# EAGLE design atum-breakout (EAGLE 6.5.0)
AUTHOR: Brad Campbell; REV: A; TITLE: Atum Breakout
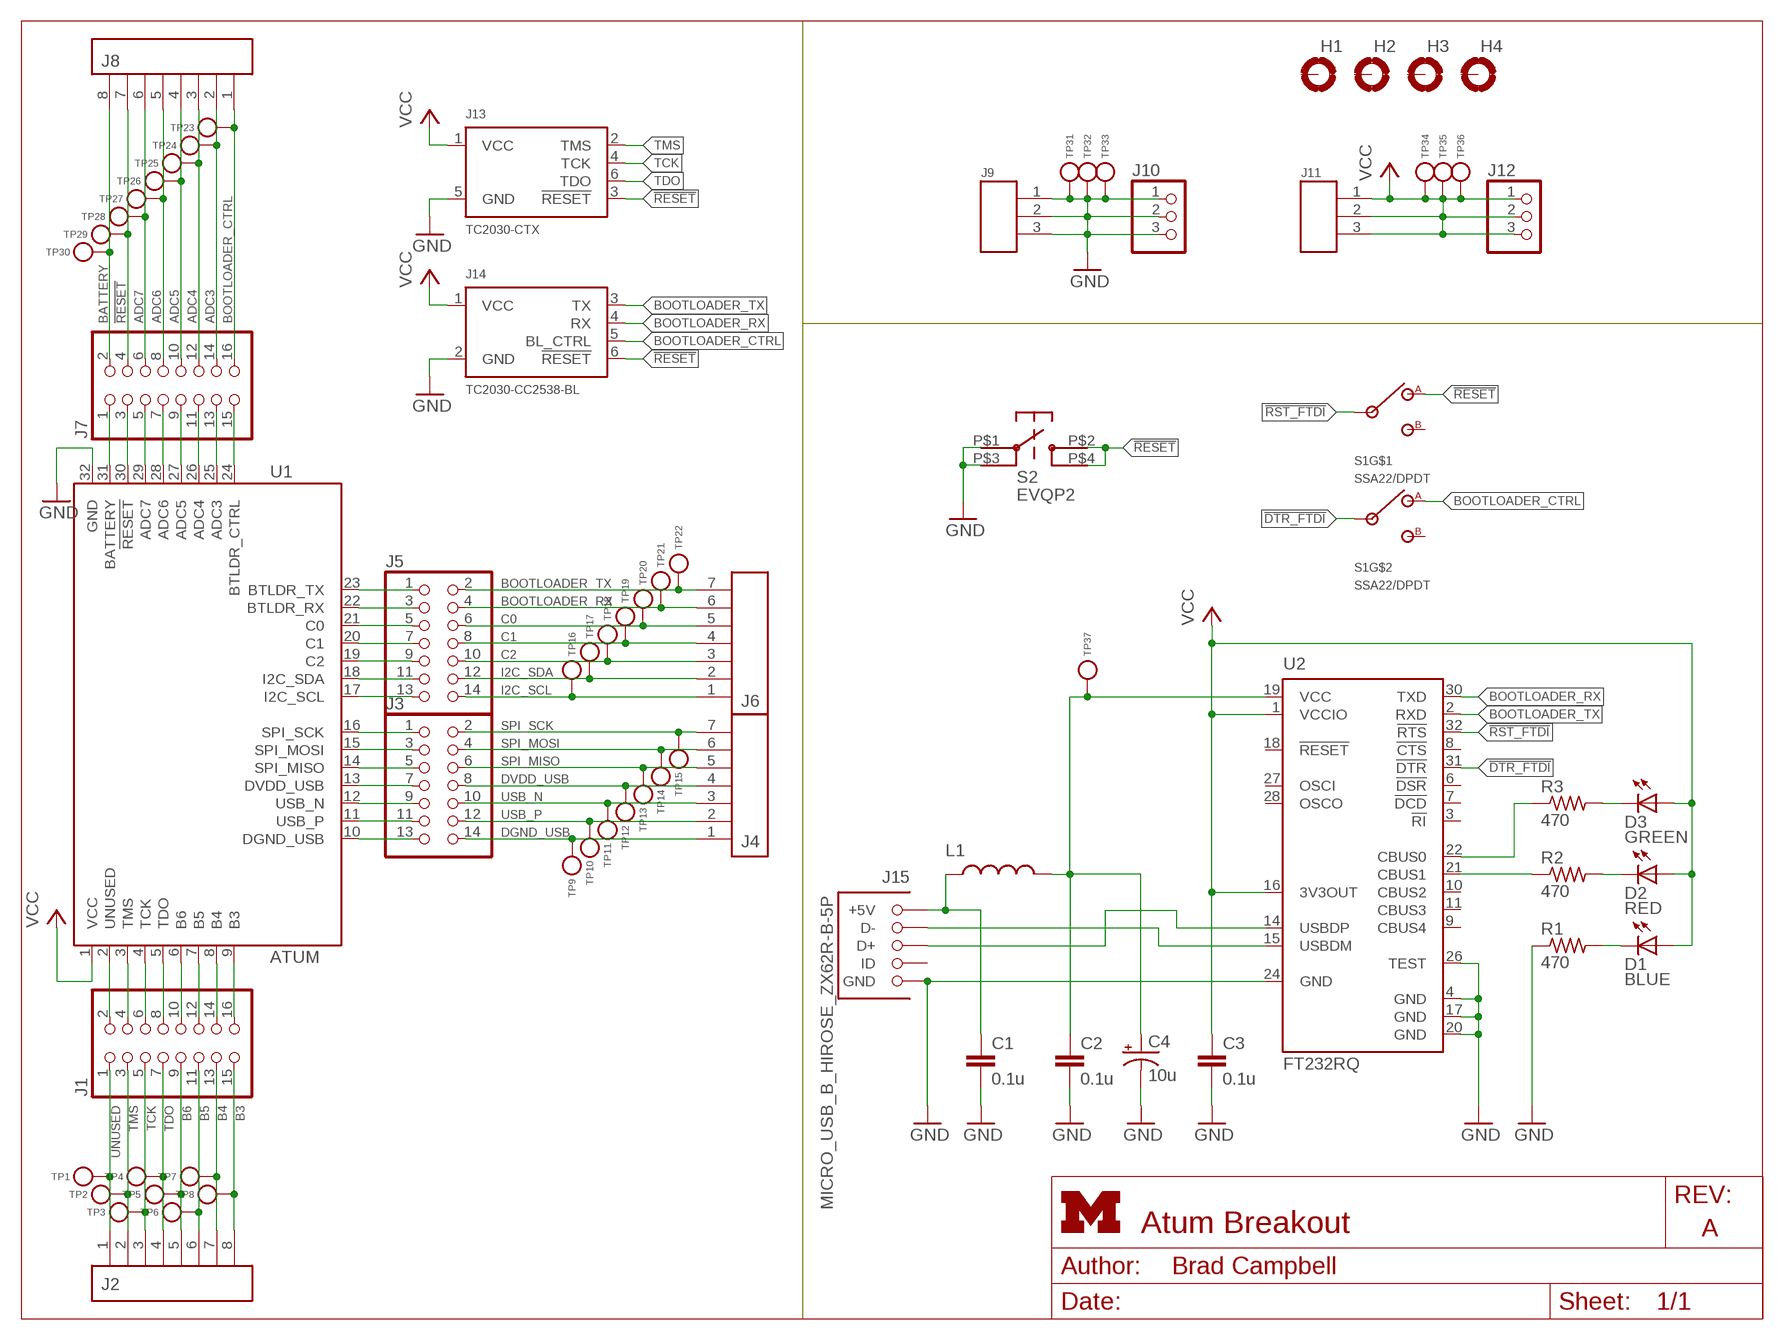
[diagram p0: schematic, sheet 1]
FRAME1 (LETTER_L): HEIGHT: 8.5in; WIDTH: 11in

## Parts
C1  0.1u  C-EUC0603  [C0603]
C2  0.1u  C-EUC0603  [C0603]
C3  0.1u  C-EUC0603  [C0603]
C4  10u  CAP_POL1206  [EIA3216]
D1  BLUE  LED0603  [LED-0603]
D2  RED  LED0603  [LED-0603]
D3  GREEN  LED0603  [LED-0603]
H1  MOUNT-PAD-ROUND3.2  [3,2-PAD]
H2  MOUNT-PAD-ROUND3.2  [3,2-PAD]
H3  MOUNT-PAD-ROUND3.2  [3,2-PAD]
H4  MOUNT-PAD-ROUND3.2  [3,2-PAD]
J1  PINHD-2X8  [2X08]
J2  SCREW-TERMINAL_8_0.100  [CONN_BLOCK_8]
J3  PINHD-2X7  [2X07]
J4  SCREW-TERMINAL_7_0.100  [CONN_BLOCK_7]
J5  PINHD-2X7  [2X07]
J6  SCREW-TERMINAL_7_0.100  [CONN_BLOCK_7]
J7  PINHD-2X8  [2X08]
J8  SCREW-TERMINAL_8_0.100  [CONN_BLOCK_8]
J9  SCREW-TERMINAL_3_0.100  [CONN_BLOCK_3]
J10  PINHD-1X3  [1X03]
J11  SCREW-TERMINAL_3_0.100  [CONN_BLOCK_3]
J12  PINHD-1X3  [1X03]
J13  TC2030-CTX  [TC2030-IDC]
J14  TC2030-CC2538-BL  [TC2030-IDC]
J15  MICRO_USB_B_HIROSE_ZX62R-B-5P  [USB_MICRO_B-HIROSE-ZX62R-B-5P]
L1  INDUCTOR0603  [0603]
R1  470  R-US_R0603  [R0603]
R2  470  R-US_R0603  [R0603]
R3  470  R-US_R0603  [R0603]
S1  SSA22/DPDT  [SSA22/DPDT]
S2  EVQP2  [EVQP2]
TP1  TEST_POINT_0.040IN  [TESTPOINT_0.040IN]
TP2  TEST_POINT_0.040IN  [TESTPOINT_0.040IN]
TP3  TEST_POINT_0.040IN  [TESTPOINT_0.040IN]
TP4  TEST_POINT_0.040IN  [TESTPOINT_0.040IN]
TP5  TEST_POINT_0.040IN  [TESTPOINT_0.040IN]
TP6  TEST_POINT_0.040IN  [TESTPOINT_0.040IN]
TP7  TEST_POINT_0.040IN  [TESTPOINT_0.040IN]
TP8  TEST_POINT_0.040IN  [TESTPOINT_0.040IN]
TP9  TEST_POINT_0.040IN  [TESTPOINT_0.040IN]
TP10  TEST_POINT_0.040IN  [TESTPOINT_0.040IN]
TP11  TEST_POINT_0.040IN  [TESTPOINT_0.040IN]
TP12  TEST_POINT_0.040IN  [TESTPOINT_0.040IN]
TP13  TEST_POINT_0.040IN  [TESTPOINT_0.040IN]
TP14  TEST_POINT_0.040IN  [TESTPOINT_0.040IN]
TP15  TEST_POINT_0.040IN  [TESTPOINT_0.040IN]
TP16  TEST_POINT_0.040IN  [TESTPOINT_0.040IN]
TP17  TEST_POINT_0.040IN  [TESTPOINT_0.040IN]
TP18  TEST_POINT_0.040IN  [TESTPOINT_0.040IN]
TP19  TEST_POINT_0.040IN  [TESTPOINT_0.040IN]
TP20  TEST_POINT_0.040IN  [TESTPOINT_0.040IN]
TP21  TEST_POINT_0.040IN  [TESTPOINT_0.040IN]
TP22  TEST_POINT_0.040IN  [TESTPOINT_0.040IN]
TP23  TEST_POINT_0.040IN  [TESTPOINT_0.040IN]
TP24  TEST_POINT_0.040IN  [TESTPOINT_0.040IN]
TP25  TEST_POINT_0.040IN  [TESTPOINT_0.040IN]
TP26  TEST_POINT_0.040IN  [TESTPOINT_0.040IN]
TP27  TEST_POINT_0.040IN  [TESTPOINT_0.040IN]
TP28  TEST_POINT_0.040IN  [TESTPOINT_0.040IN]
TP29  TEST_POINT_0.040IN  [TESTPOINT_0.040IN]
TP30  TEST_POINT_0.040IN  [TESTPOINT_0.040IN]
TP31  TEST_POINT_0.040IN  [TESTPOINT_0.040IN]
TP32  TEST_POINT_0.040IN  [TESTPOINT_0.040IN]
TP33  TEST_POINT_0.040IN  [TESTPOINT_0.040IN]
TP34  TEST_POINT_0.040IN  [TESTPOINT_0.040IN]
TP35  TEST_POINT_0.040IN  [TESTPOINT_0.040IN]
TP36  TEST_POINT_0.040IN  [TESTPOINT_0.040IN]
TP37  TEST_POINT_0.040IN  [TESTPOINT_0.040IN]
U1  ATUM  [ATUM]
U2  FT232RQ  [QFN32]

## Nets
!DTR_FTDI: S1.COM2 U2.31(!DTR)
!RESET: J7.3 J7.4 J8.7 J13.3(!RESET) J14.6(!RESET) S1.A1 S2.P$2 S2.P$4 TP29.TESTPOINT U1.30(!RESET)
!RST_FTDI: S1.COM1 U2.32(!RTS)
ADC3: J7.13 J7.14 J8.2 TP24.TESTPOINT U1.25(ADC3)
ADC4: J7.11 J7.12 J8.3 TP25.TESTPOINT U1.26(ADC4)
ADC5: J7.9 J7.10 J8.4 TP26.TESTPOINT U1.27(ADC5)
ADC6: J7.7 J7.8 J8.5 TP27.TESTPOINT U1.28(ADC6)
ADC7: J7.5 J7.6 J8.6 TP28.TESTPOINT U1.29(ADC7)
B3: J1.15 J1.16 J2.8 TP8.TESTPOINT U1.9(B3)
B4: J1.13 J1.14 J2.7 TP7.TESTPOINT U1.8(B4)
B5: J1.11 J1.12 J2.6 TP6.TESTPOINT U1.7(B5)
B6: J1.9 J1.10 J2.5 TP5.TESTPOINT U1.6(B6)
BATTERY: J7.1 J7.2 J8.8 TP30.TESTPOINT U1.31(BATTERY)
BOOTLOADER_CTRL: J7.15 J7.16 J8.1 J14.5(BL_CTRL) S1.A2 TP23.TESTPOINT U1.24(BTLDR_CTRL)
BOOTLOADER_RX: J5.3 J5.4 J6.6 J14.4(RX) TP21.TESTPOINT U1.22(BTLDR_RX) U2.30(TXD)
BOOTLOADER_TX: J5.1 J5.2 J6.7 J14.3(TX) TP22.TESTPOINT U1.23(BTLDR_TX) U2.2(RXD)
C0: J5.5 J5.6 J6.5 TP20.TESTPOINT U1.21(C0)
C1: J5.7 J5.8 J6.4 TP19.TESTPOINT U1.20(C1)
C2: J5.9 J5.10 J6.3 TP18.TESTPOINT U1.19(C2)
DGND_USB: J3.13 J3.14 J4.1 TP9.TESTPOINT U1.10(DGND_USB)
DVDD_USB: J3.7 J3.8 J4.4 TP12.TESTPOINT U1.13(DVDD_USB)
GND: C1.2 C2.2 C3.2 C4.C(-) J9.1 J9.2 J9.3 J10.1 J10.2 J10.3 J13.5(GND) J14.2(GND) J15.5(GND) R1.1 S2.P$1 S2.P$3 TP31.TESTPOINT TP32.TESTPOINT TP33.TESTPOINT U1.32(GND) U2.4(GND) U2.17(GND) U2.20(GND) U2.24(GND) U2.26(TEST)
I2C_SCL: J5.13 J5.14 J6.1 TP16.TESTPOINT U1.17(I2C_SCL)
I2C_SDA: J5.11 J5.12 J6.2 TP17.TESTPOINT U1.18(I2C_SDA)
N$1: R3.1 U2.22(CBUS0)
N$2: D2.C R2.2
N$3: J15.2(D-) U2.15(USBDM)
N$4: J15.3(D+) U2.14(USBDP)
N$5: R2.1 U2.21(CBUS1)
N$6: C2.1 C4.A(+) L1.2 TP37.TESTPOINT U2.19(VCC)
N$7: D3.C R3.2
N$8: D1.C R1.2
SPI_MISO: J3.5 J3.6 J4.5 TP13.TESTPOINT U1.14(SPI_MISO)
SPI_MOSI: J3.3 J3.4 J4.6 TP14.TESTPOINT U1.15(SPI_MOSI)
SPI_SCK: J3.1 J3.2 J4.7 TP15.TESTPOINT U1.16(SPI_SCK)
TCK: J1.5 J1.6 J2.3 J13.4(TCK) TP3.TESTPOINT U1.4(TCK)
TDO: J1.7 J1.8 J2.4 J13.6(TDO) TP4.TESTPOINT U1.5(TDO)
TMS: J1.3 J1.4 J2.2 J13.2(TMS) TP2.TESTPOINT U1.3(TMS)
UNUSED: J1.1 J1.2 J2.1 TP1.TESTPOINT U1.2(UNUSED)
USB5V: C1.1 J15.1(+5V) L1.1
USB_N: J3.9 J3.10 J4.3 TP11.TESTPOINT U1.12(USB_N)
USB_P: J3.11 J3.12 J4.2 TP10.TESTPOINT U1.11(USB_P)
VCC: C3.1 D1.A D2.A D3.A J11.1 J11.2 J11.3 J12.1 J12.2 J12.3 J13.1(VCC) J14.1(VCC) TP34.TESTPOINT TP35.TESTPOINT TP36.TESTPOINT U1.1(VCC) U2.1(VCCIO) U2.16(3V3OUT)
Unconnected: H1.B3,2(MOUNT) H2.B3,2(MOUNT) H3.B3,2(MOUNT) H4.B3,2(MOUNT) J15.4(ID) S1.B1 S1.B2 U2.3(!RI) U2.6(!DSR) U2.7(!DCD) U2.8(!CTS) U2.9(CBUS4) U2.10(CBUS2) U2.11(CBUS3) U2.18(!RESET) U2.27(OSCI) U2.28(OSCO)

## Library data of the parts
C1-C3 = rcl:C-EU: CAPACITOR, European symbol; DIGIKEY: 445-1316-1-ND
C4 = SparkFun:CAP_POL: Capacitor Polarized; DIGIKEY: 478-1655-1-ND
D1-D3 = SparkFun:LED: LEDs
H1-H4 = holes:MOUNT-PAD-ROUND: MOUNTING PAD, round
J1 J7 = pinhead:PINHD-2X8: PIN HEADER; DIGIKEY: 609-3364-ND; MOUSER: 649-68602-116HLF; NEWARK: 20M2833
J2 J8 = headers:SCREW-TERMINAL_8_0.100: 8x 0.100 in screw terminal block; DIGIKEY: 277-1279-ND
J3 J5 = pinhead:PINHD-2X7: PIN HEADER; DIGIKEY: 609-3491-ND; MOUSER: 649-67996-114HLF; NEWARK: 30M1973
J4 J6 = headers:SCREW-TERMINAL_7_0.100: 7x 0.100 in screw terminal block; DIGIKEY: 277-1278-ND
J9 J11 = headers:SCREW-TERMINAL_3_0.100: 3x 0.100 in screw terminal block; DIGIKEY: 277-1274-ND
J10 J12 = pinhead:PINHD-1X3: PIN HEADER
J13 = connector:TC2030-CTX: Tag Connect footprint for ARM JTAG. 10 pin ARM Cortex Debug Connector.
J14 = connector:TC2030-CC2538-BL: Tag connect programmer for the CC2538 bootloader. The RX/TX switch happens on the programmer board, so when using this connect the TX pin to the TX pin on the CC2538 and same for the RX.
J15 = connector:MICRO_USB_B_HIROSE_ZX62R-B-5P: USB Micro B Connector Rounded side is up.; DIGIKEY: H11574CT-ND; MOUSER: 798-ZX62R-B-5P; NEWARK: 69W0714
L1 = SparkFun:INDUCTOR: Inductors; DIGIKEY: 240-2373-1-ND
R1-R3 = rcl:R-US_: RESISTOR, American symbol
S1 = switches:SSA22/DPDT: SW SLIDE DPDT 2POS SSA SER 30V; DIGIKEY: 450-1604-ND; MOUSER: 506-SSA22; NEWARK: 50F5561
S2 = berkeley-epic:EVQP2; DIGIKEY: P11084SCT-ND; MOUSER: 667-EVQ-P2K02Q
TP1-TP37 = headers:TEST_POINT_0.040IN: 0.040in Test Point; DIGIKEY: 5001K-ND
U1 = atum:ATUM: Atum sensorboard prototyping module.
U2 = ftdichip:FT232R: Source: http://www.ftdichip.com/Documents/DataSheets/DS_FT232R_v104.pdf; DIGIKEY: 768-1008-1-ND; MPN: FT232RQ; OC_FARNELL: 1146033; OC_NEWARK: 91K9919

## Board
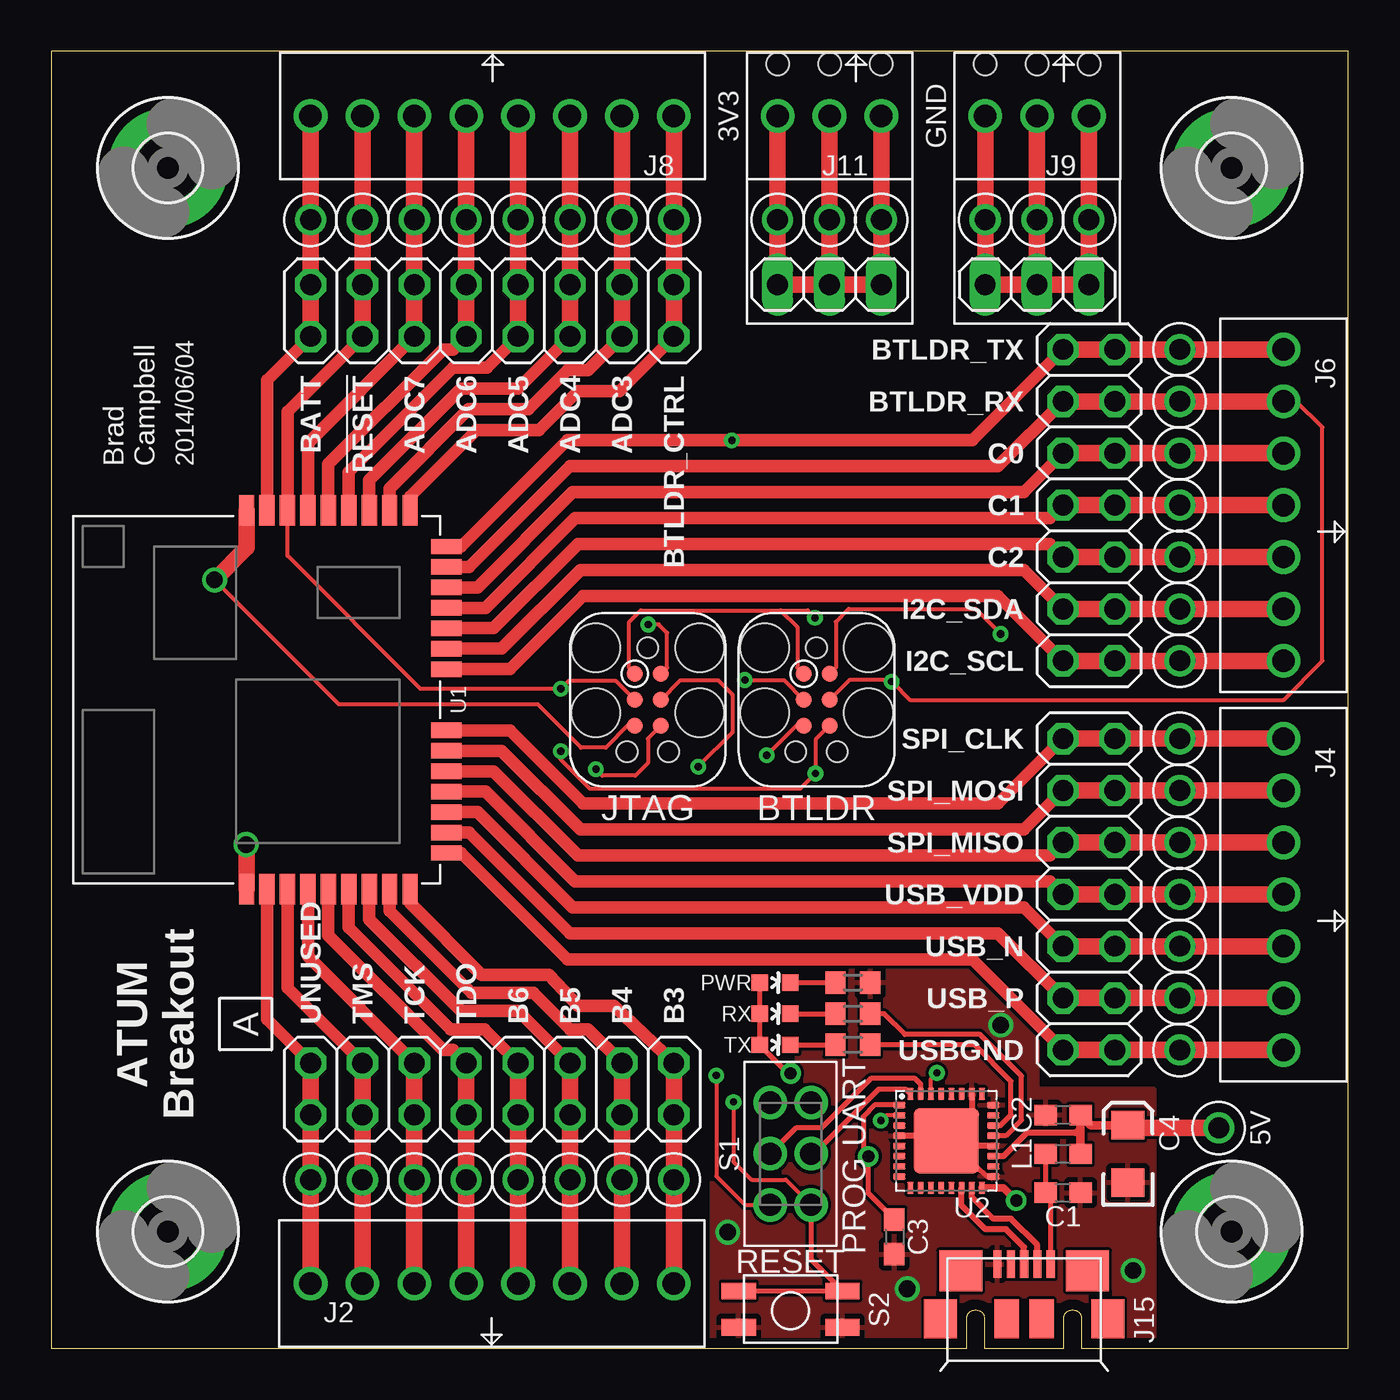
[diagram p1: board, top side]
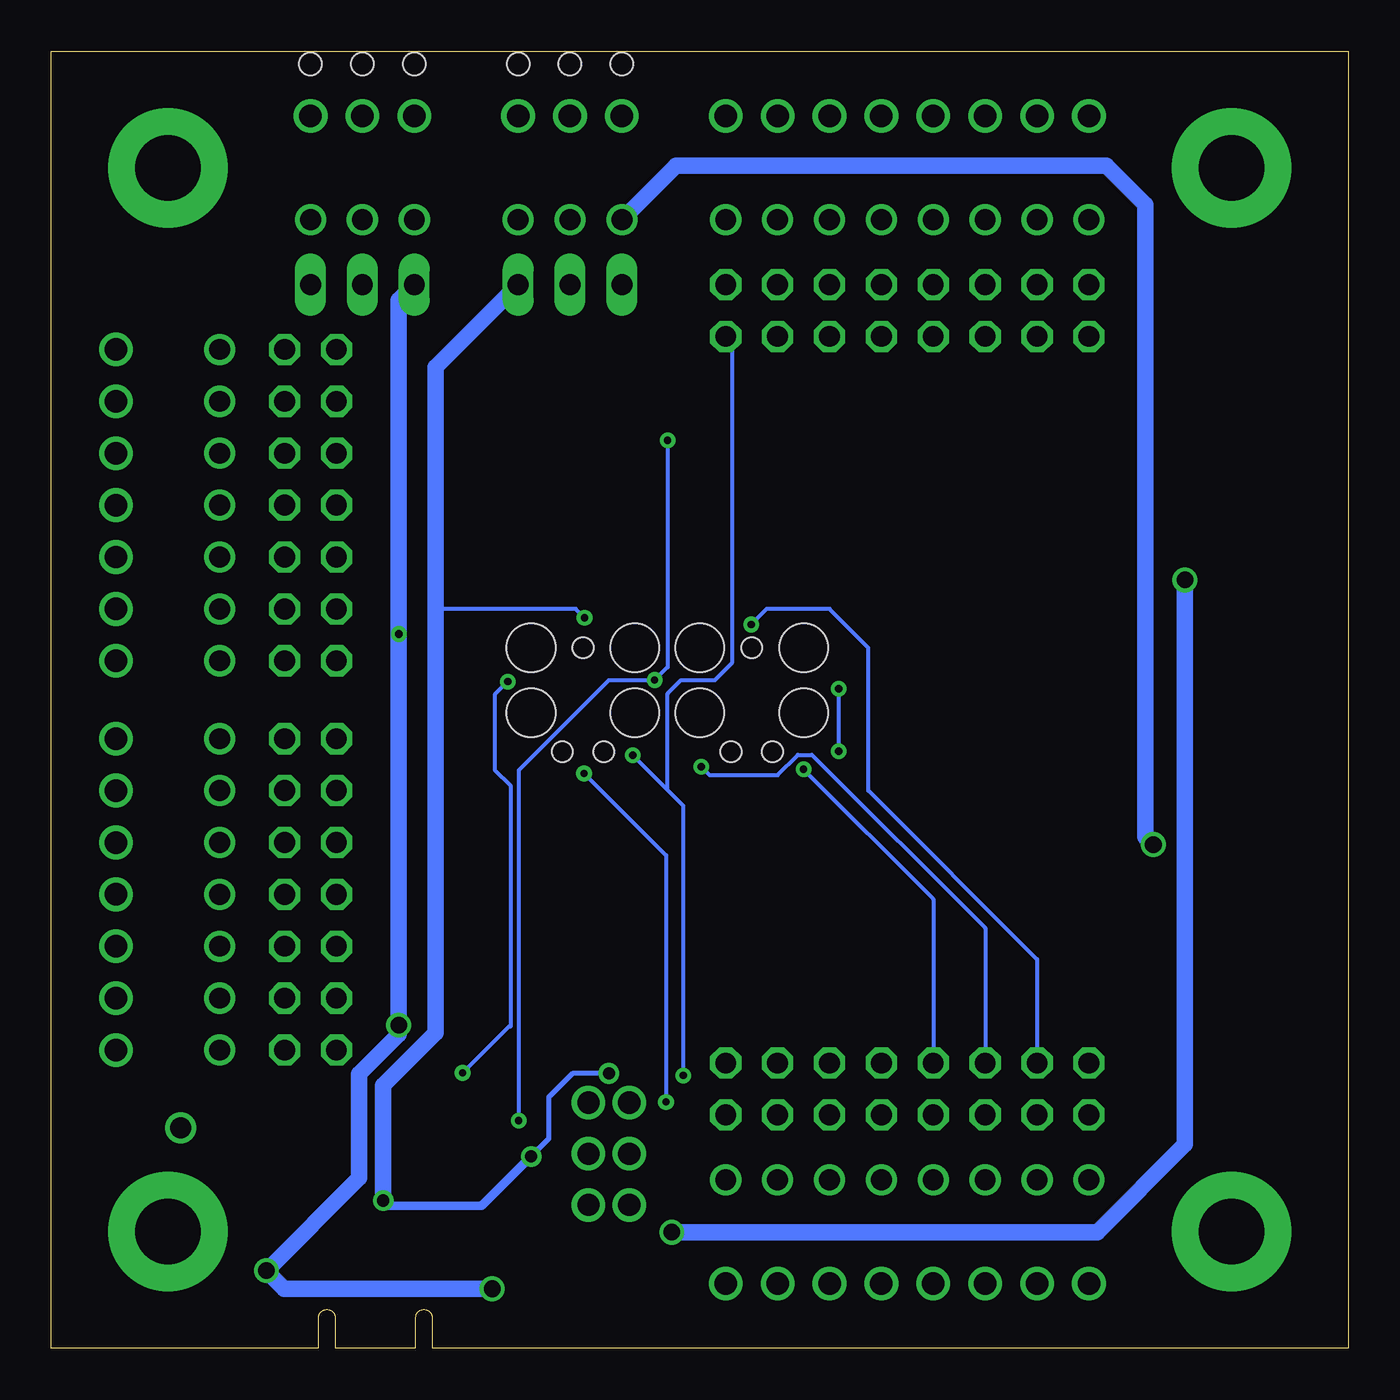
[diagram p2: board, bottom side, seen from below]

Size 63.5 x 63.5 mm. Coordinates in mm from the lower left corner, seen from the top.
Outline: 52.7,0 63.5,0 63.5,63.5 0,63.5 0,0 42.55,0
Copper layers (1*16): Top 0.0178mm / dielectric 59mil / Bottom 0.0178mm
Design rules "sunstone-2lyr_v1.0.0.3 *": minimum track width 6mil, minimum drill 14mil, track to track 6mil, track to pad 6mil, pad to pad 6mil, via to via 6mil, smd to smd 6mil, copper to edge 20mil, drill to drill 16mil, minimum pad ring 8mil, minimum via ring 8mil, stop-mask expansion 3mil, vias tented up to drill 40mil, thermal gap 10mil

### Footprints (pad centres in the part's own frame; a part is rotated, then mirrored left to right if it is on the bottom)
C0603 = smd 1.1 x 1: 1 -0.85,0; 2 0.85,0
EIA3216 = smd 1.4 x 1.6: A 1.4,0; C -1.4,0
LED-0603 = smd 0.8 x 0.8: A 0,-0.75; C 0,0.75
3,2-PAD = drill 3.2 pad 5.842: B3,2 0,0
2X08 = drill 1.016 octagon: 1 -8.89,-1.27; 2 -8.89,1.27; 3 -6.35,-1.27; 4 -6.35,1.27; 5 -3.81,-1.27; 6 -3.81,1.27; 7 -1.27,-1.27; 8 -1.27,1.27; 9 1.27,-1.27; 10 1.27,1.27; 11 3.81,-1.27; 12 3.81,1.27; 13 6.35,-1.27; 14 6.35,1.27; 15 8.89,-1.27; 16 8.89,1.27
CONN_BLOCK_8 = drill 1.1: 1 -8.89,0; 2 -6.35,0; 3 -3.81,0; 4 -1.27,0; 5 1.27,0; 6 3.81,0; 7 6.35,0; 8 8.89,0
2X07 = drill 1.016 octagon: 1 -7.62,-1.27; 2 -7.62,1.27; 3 -5.08,-1.27; 4 -5.08,1.27; 5 -2.54,-1.27; 6 -2.54,1.27; 7 0,-1.27; 8 0,1.27; 9 2.54,-1.27; 10 2.54,1.27; 11 5.08,-1.27; 12 5.08,1.27; 13 7.62,-1.27; 14 7.62,1.27
CONN_BLOCK_7 = drill 1.1: 1 -7.62,0; 2 -5.08,0; 3 -2.54,0; 4 0,0; 5 2.54,0; 6 5.08,0; 7 7.62,0
CONN_BLOCK_3 = drill 1.1: 1 -2.54,0; 2 0,0; 3 2.54,0 | hole 1.1: -2.54,-2.54; 0,-2.54; 2.54,-2.54
1X03 = drill 1.016 long: 1 -2.54,0; 2 0,0; 3 2.54,0
TC2030-IDC = smd 0.787 x 0.787: 1 -1.27,-0.635; 2 -1.27,0.635; 3 0,-0.635; 4 0,0.635; 5 1.27,-0.635; 6 1.27,0.635 | hole 2.375: -2.54,2.54; 0.635,2.54; 0.635,-2.54; -2.54,-2.54 | hole 1.016: -2.54,0; 2.54,1.016; 2.54,-1.016
USB_MICRO_B-HIROSE-ZX62R-B-5P = smd 0.4 x 1.35: 1 1.3,4.125; 2 0.65,4.125; 3 0,4.125; 4 -0.65,4.125; 5 -1.3,4.125 | smd 2.1 x 2: P$1 3.1,3.8; P$2 -3.1,3.8 | smd 1.6 x 1.9: P$3 -4.1,1.45; P$6 4.1,1.45 | smd 1.2 x 1.9: P$4 -0.85,1.45; P$5 0.85,1.45
0603 = smd 1.1 x 1: 1 -0.85,0; 2 0.85,0
R0603 = smd 1 x 1.1: 1 -0.85,0; 2 0.85,0
SSA22/DPDT = drill 1.092: A1 2.5,1; A2 2.5,-1; B1 -2.5,1; B2 -2.5,-1; COM1 0,1; COM2 0,-1
EVQP2 = smd 1.676 x 0.813: P$1 -2.54,-0.87; P$2 -2.54,0.908; P$3 2.54,-0.87; P$4 2.54,0.908
TESTPOINT_0.040IN = drill 1.016: TESTPOINT 0,0
ATUM = smd 0.754 x 1.5: 1 -9.479,-9.279; 2 -8.479,-9.279; 3 -7.479,-9.279; 4 -6.479,-9.279; 5 -5.479,-9.279; 6 -4.479,-9.279; 7 -3.479,-9.279; 8 -2.479,-9.279; 9 -1.479,-9.279; 24 -1.479,9.279; 25 -2.479,9.279; 26 -3.479,9.279; 27 -4.479,9.279; 28 -5.479,9.279; 29 -6.479,9.279; 30 -7.479,9.279; 31 -8.479,9.279; 32 -9.479,9.279 | smd 1.5 x 0.754: 10 0.3,-7.5; 11 0.3,-6.5; 12 0.3,-5.5; 13 0.3,-4.5; 14 0.3,-3.5; 15 0.3,-2.5; 16 0.3,-1.5; 17 0.3,1.5; 18 0.3,2.5; 19 0.3,3.5; 20 0.3,4.5; 21 0.3,5.5; 22 0.3,6.5; 23 0.3,7.5
QFN32 = smd 0.6 x 0.3: 1 -2.3,1.75; 2 -2.3,1.25; 3 -2.3,0.75; 4 -2.3,0.25; 5 -2.3,-0.25; 6 -2.3,-0.75; 7 -2.3,-1.25; 8 -2.3,-1.75; 17 2.3,-1.75; 18 2.3,-1.25; 19 2.3,-0.75; 20 2.3,-0.25; 21 2.3,0.25; 22 2.3,0.75; 23 2.3,1.25; 24 2.3,1.75 | smd 0.3 x 0.6: 9 -1.75,-2.3; 10 -1.25,-2.3; 11 -0.75,-2.3; 12 -0.25,-2.3; 13 0.25,-2.3; 14 0.75,-2.3; 15 1.25,-2.3; 16 1.75,-2.3; 25 1.75,2.3; 26 1.25,2.3; 27 0.75,2.3; 28 0.25,2.3; 29 -0.25,2.3; 30 -0.75,2.3; 31 -1.25,2.3; 32 -1.75,2.3 | smd 3.2 x 3.2: EXP 0,0

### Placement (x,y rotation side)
C1  49.53,7.62 0 top
C2  49.53,11.43 180 top
C3  41.27,5.46 270 top
C4  52.7,9.53 90 top
D1  35.43,17.91 270 top
D2  35.43,16.38 270 top
D3  35.43,14.86 270 top
H1  57.78,5.71 0 top
H2  5.71,5.71 0 top
H3  57.78,57.78 0 top
H4  5.71,57.78 0 top
J1  21.59,12.7 0 top
J2  21.59,3.17 0 top
J3  50.8,22.23 270 top
J4  60.33,22.23 90 top
J5  50.8,41.27 270 top
J6  60.33,41.27 90 top
J7  21.59,50.8 0 top
J8  21.59,60.33 180 top
J9  48.26,60.33 180 top
J10  48.26,52.07 0 top
J11  38.1,60.33 180 top
J12  38.1,52.07 0 top
J13  29.21,31.75 270 top
J14  37.47,31.75 270 top
J15  47.62,0 0 top
L1  49.53,9.53 0 top
R1  39.24,17.91 180 top
R2  39.24,16.38 180 top
R3  39.24,14.86 180 top
S1  36.2,9.53 270 top
S2  36.2,1.91 0 top
TP1  12.7,8.26 0 top
TP2  15.24,8.26 0 top
TP3  17.78,8.26 0 top
TP4  20.32,8.26 0 top
TP5  22.86,8.26 0 top
TP6  25.4,8.26 0 top
TP7  27.94,8.26 0 top
TP8  30.48,8.26 0 top
TP9  55.24,14.61 0 top
TP10  55.24,17.14 0 top
TP11  55.24,19.68 0 top
TP12  55.24,22.23 0 top
TP13  55.24,24.77 0 top
TP14  55.24,27.3 0 top
TP15  55.24,29.84 0 top
TP16  55.24,33.66 0 top
TP17  55.24,36.2 0 top
TP18  55.24,38.73 0 top
TP19  55.24,41.27 0 top
TP20  55.24,43.81 0 top
TP21  55.24,46.35 0 top
TP22  55.24,48.9 0 top
TP23  30.48,55.24 0 top
TP24  27.94,55.24 0 top
TP25  25.4,55.24 0 top
TP26  22.86,55.24 0 top
TP27  20.32,55.24 0 top
TP28  17.78,55.24 0 top
TP29  15.24,55.24 0 top
TP30  12.7,55.24 0 top
TP31  50.8,55.24 0 top
TP32  48.26,55.24 0 top
TP33  45.72,55.24 0 top
TP34  40.64,55.24 0 top
TP35  38.1,55.24 0 top
TP36  35.56,55.24 0 top
TP37  57.15,10.79 0 top
U1  19.05,31.75 0 top
U2  43.81,10.16 0 top

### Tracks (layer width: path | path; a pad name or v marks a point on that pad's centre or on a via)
!DTR_FTDI
  Top 0.254: U2.31 42.56,12.93 42.29,13.21 40.13,13.21 37.72,10.79 36.47,10.79 S1.COM2
!RESET  (via drill 0.36)
  Top 0.203: J13.3 27.66,32.66 25.32,32.66 v24.94,32.28 18.09,32.28 11.57,38.8 U1.30 | J14.6 37.41,29.79 v37.41,28.14 36.68,27.41 26.36,27.41 24.94,28.83 v24.94,29.23 | v33.4,12.06 33.4,9.14 34.29,8.26 35.97,8.26 S1.A1
  Top 0.254: S2.P$2 S2.P$4 37.2,4.35 S1.A1
  Top 0.61: U1.30 11.57,45.86 J7.3
  Top 0.813: J7.3 J7.4 TP29.TESTPOINT J8.7
  Bottom 0.203: v37.41,28.14 33.4,24.13 v33.4,12.06 | v24.94,29.23 v24.94,32.28
!RST_FTDI
  Top 0.254: S1.COM1 37.34,9.53 40.51,12.7 41.83,12.7 U2.32
ADC3
  Top 0.61: U1.25 16.57,42.1 20.45,45.97 23.37,45.97 25.27,47.88 26.29,47.88 J7.13
  Top 0.813: J8.2 TP24.TESTPOINT J7.14 J7.13
ADC4
  Top 0.61: U1.26 15.57,42.49 20.07,46.99 22.86,46.99 J7.11
  Top 0.813: J7.11 J7.12 TP25.TESTPOINT J8.3
ADC5
  Top 0.61: U1.27 14.57,42.89 19.68,48.01 21.34,48.01 J7.9
  Top 0.813: J8.4 TP26.TESTPOINT J7.10 J7.9
ADC6
  Top 0.61: U1.28 13.57,43.29 19.18,48.9 19.68,48.9 J7.7
  Top 0.813: J7.7 J7.8 TP27.TESTPOINT J8.5
ADC7
  Top 0.61: U1.29 12.57,44.32 J7.5
  Top 0.813: J8.6 TP28.TESTPOINT J7.6 J7.5
B3
  Top 0.61: U1.9 17.57,21.8 21.08,18.29 24.38,18.29 25.78,16.76 27.56,16.76 J1.16
  Top 0.813: J2.8 TP8.TESTPOINT J1.15 J1.16
B4
  Top 0.61: U1.8 16.57,21.4 20.57,17.4 23.62,17.4 25.4,15.62 26.29,15.62 J1.14
  Top 0.813: J1.14 J1.13 TP7.TESTPOINT J2.7
B5
  Top 0.61: U1.7 15.57,21 20.07,16.51 22.86,16.51 J1.12
  Top 0.813: J2.6 TP6.TESTPOINT J1.11 J1.12
B6
  Top 0.61: U1.6 14.57,20.61 19.56,15.62 21.21,15.62 J1.10
  Top 0.813: J1.10 J1.9 TP5.TESTPOINT J2.5
BATTERY
  Top 0.61: U1.31 10.57,47.4 J7.1
  Top 0.813: J8.8 TP30.TESTPOINT J7.2 J7.1
BOOTLOADER_CTRL  (via drill 0.36)
  Top 0.203: J14.5 36.47,30.48 v35.03,29.03 | v32.56,13.36 32.56,8.43 33.97,7.03 S1.A2
  Top 0.61: U1.24 17.57,41.7 20.83,44.96 23.88,44.96 25.78,46.86 27.81,46.86 J7.15
  Top 0.813: J7.15 J7.16 TP23.TESTPOINT J8.1
  Bottom 0.203: v35.03,29.03 33.33,27.33 | 33.33,27.33 32.56,26.57 v32.56,13.36 | 33.33,27.33 33.33,32.05 32.66,32.72 31.01,32.72 30.15,33.58 30.15,49.2 J7.15
BOOTLOADER_RX  (via drill 0.36)
  Top 0.203: U2.30 43.06,13.2 v43.36,13.49 | J14.4 39.06,32.72 41.07,32.72 v41.15,32.64 42.04,31.75 60.33,31.75 62.23,33.66 62.23,45.09 60.96,46.35 J6.6
  Top 0.61: U1.22 20.47,38.25 25.4,43.18 46.35,43.18 J5.3
  Top 0.813: J5.3 J5.4 TP21.TESTPOINT J6.6
  Bottom 0.203: v41.15,32.64 41.78,32 41.78,28.32 41.02,27.56 41.02,15.75 41.1,15.75 v43.36,13.49
BOOTLOADER_TX  (via drill 0.36)
  Top 0.203: U2.2 40.9,11.41 v40.62,11.15 | v33.96,32.72 35.87,32.72 J14.3
  Top 0.61: U1.23 20.07,39.25 25.27,44.45 v33.33,44.45 45.09,44.45 J5.1
  Top 0.813: J6.7 TP22.TESTPOINT J5.2 J5.1
  Bottom 0.203: v40.62,11.15 40.62,28.3 36.2,32.72 v33.96,32.72 33.33,33.35 v33.33,44.45
C0
  Top 0.61: U1.21 20.87,37.25 25.53,41.91 47.62,41.91 J5.5
  Top 0.813: J6.5 TP20.TESTPOINT J5.6 J5.5
C1
  Top 0.61: U1.20 21.26,36.25 25.65,40.64 48.9,40.64 J5.7
  Top 0.813: J5.7 J5.8 TP19.TESTPOINT J6.4
C2
  Top 0.61: U1.19 21.66,35.25 25.78,39.37 48.9,39.37 J5.9
  Top 0.813: J5.9 J5.10 TP18.TESTPOINT J6.3
DGND_USB
  Top 0.61: U1.10 20.07,24.25 25.27,19.05 45.09,19.05 J3.13
  Top 0.813: J3.13 J3.14 TP9.TESTPOINT J4.1
DVDD_USB
  Top 0.61: U1.13 21.26,27.25 25.65,22.86 48.9,22.86 J3.7
  Top 0.813: J3.7 J3.8 TP12.TESTPOINT J4.4
GND  (via drill 0.36, 0.81)
  Top 0.203: J13.5 28.22,30.48 27.15,29.41 25.93,29.41 23.82,31.52 14.1,31.52 v8,37.62 | J14.2 38.41,33.33 38.41,35.56 39.04,36.2 45.26,36.2 v46.48,34.98
  Top 0.254: U2.17 45.82,8.41 45.47,8.71 44.96,9.22 44.96,9.78
  Top 0.305: U2.26 45.06,11.66 43.81,10.41 | 43.81,10.41 U2.4 | U2.20 45.09,9.91 | 45.09,9.91 44.31,9.91 43.81,10.41 | 44.96,9.78 45.09,9.91
  Top 0.813: J9.3 TP33.TESTPOINT J10.1 | J9.2 TP32.TESTPOINT J10.2 J10.1 | J9.1 TP31.TESTPOINT J10.3 J10.1 | v8,37.62 9.57,39.19 U1.32
  Bottom 0.813: J10.1 46.48,51.31 v46.48,34.98 v46.48,34.95 v46.48,15.82 46.48,15.37 48.41,13.44 48.41,8.36 v52.96,3.81 | v8,37.62 8,9.98 12.29,5.69 v33.12,5.69 | v41.91,2.92 52.09,2.92 52.96,3.79
  pour Top: 32.38,0 32.38,20.32 48.26,20.32 48.26,12.7 53.98,12.7 53.98,0
I2C_SCL
  Top 0.61: J5.13 46.35,36.83 26.04,36.83 22.45,33.25 U1.17
  Top 0.813: J5.13 J5.14 TP16.TESTPOINT J6.1
I2C_SDA
  Top 0.61: J5.11 47.62,38.1 25.91,38.1 22.06,34.25 U1.18
  Top 0.813: J6.2 TP17.TESTPOINT J5.12 J5.11
N$1
  Top 0.254: U2.22 46.47,10.91 46.99,11.43 46.99,13.08 45.21,14.86 R3.1
N$2
  Top 0.254: D2.C R2.2
N$3
  Top 0.305: J15.2 48.27,5.07 46.99,6.35 46.1,6.35 45.06,7.39 U2.15
N$4
  Top 0.305: J15.3 47.62,4.95 46.74,5.84 45.72,5.84 44.56,7 U2.14
N$5
  Top 0.254: U2.21 46.73,10.41 47.5,11.18 47.5,13.34 45.47,15.37 41.78,15.37 40.77,16.38 R2.1
N$6
  Top 0.305: U2.19 46.62,9.41 47.75,10.54 50.13,10.54 50.38,10.79
  Top 0.406: C4.A 50.88,10.93 C2.1 50.38,10.79 L1.2
  Top 0.813: TP37.TESTPOINT 52.84,10.79 C4.A
N$7
  Top 0.254: D3.C R3.2
N$8
  Top 0.254: D1.C R1.2
SPI_MISO
  Top 0.61: U1.14 21.66,28.25 25.78,24.13 48.9,24.13 J3.5
  Top 0.813: J4.5 TP13.TESTPOINT J3.6 J3.5
SPI_MOSI
  Top 0.61: J3.3 47.62,25.4 25.91,25.4 22.06,29.25 U1.15
  Top 0.813: J3.3 J3.4 TP14.TESTPOINT J4.6
SPI_SCK
  Top 0.61: J3.1 46.35,26.67 26.04,26.67 22.45,30.25 U1.16
  Top 0.813: J4.7 TP15.TESTPOINT J3.2 J3.1
TCK  (via drill 0.36)
  Top 0.203: J13.4 30.81,32.72 32.64,32.72 33.35,32 33.35,30.15 v31.67,28.47
  Top 0.61: U1.4 12.57,19.18 J1.6
  Top 0.813: J1.6 J1.5 TP3.TESTPOINT J2.3
  Bottom 0.203: J1.6 17.78,20.57 26.26,29.06 26.95,29.06 27.94,28.07 31.27,28.07 v31.67,28.47
TDO  (via drill 0.36)
  Top 0.203: J13.6 29.21,29.84 29.21,28.65 28.6,28.04 26.98,28.04 v26.67,28.35
  Top 0.61: U1.5 13.57,20.21 19.18,14.61 19.68,14.61 J1.8
  Top 0.813: J2.4 TP4.TESTPOINT J1.7 J1.8
  Bottom 0.203: J1.8 20.32,22 v26.67,28.35
TMS  (via drill 0.36)
  Top 0.203: J13.2 30.15,33.33 30.15,35.03 29.74,35.43 v29.23,35.43
  Top 0.61: U1.3 11.57,17.64 J1.4
  Top 0.813: J2.2 TP2.TESTPOINT J1.3 J1.4
  Bottom 0.203: J1.4 15.24,19.05 23.5,27.3 23.5,34.29 25.4,36.2 28.47,36.2 v29.23,35.43
UNUSED
  Top 0.61: U1.2 10.57,16.1 J1.2
  Top 0.813: J1.2 J1.1 TP1.TESTPOINT J2.1
USB5V
  Top 0.254: J15.1 48.92,7.38 C1.1 L1.1
USB_N
  Top 0.61: U1.12 20.87,26.25 25.53,21.59 47.62,21.59 J3.9
  Top 0.813: J3.9 J3.10 TP11.TESTPOINT J4.3
USB_P
  Top 0.61: U1.11 20.47,25.25 25.4,20.32 46.35,20.32 J3.11
  Top 0.813: J4.2 TP10.TESTPOINT J3.12 J3.11
VCC  (via drill 0.36, 0.6, 0.81)
  Top 0.203: J13.1 28.3,33.3 28.3,35.56 28.85,36.12 35.71,36.12 | 35.71,36.12 36.52,35.31 36.52,33.33 J14.1 | 35.71,36.12 37.03,36.12 v37.39,35.76
  Top 0.254: D1.A D2.A D3.A 36.08,13.46 v36.2,13.46 | U2.1 40.31,11.91 39.75,11.35 39.75,9.65 v40.01,9.4 40.01,7.58 C3.1
  Top 0.356: U2.16 46.62,7.86 v47.24,7.24
  Top 0.813: J12.1 TP36.TESTPOINT J11.3 | J11.1 TP34.TESTPOINT J12.3 J12.1 | J11.2 TP35.TESTPOINT J12.2 J12.1 | v9.55,24.66 9.57,24.64 U1.1
  Bottom 0.203: v37.39,35.76 37.82,36.2 44.68,36.2
  Bottom 0.254: v36.2,13.46 37.97,13.46 39.14,12.29 39.14,10.26 v40.01,9.4
  Bottom 0.406: v40.01,9.4 42.42,6.99 46.99,6.99 v47.24,7.24
  Bottom 0.813: v47.24,7.24 47.24,12.88 44.68,15.44 44.68,36.2 44.68,48.03 J12.3 | TP36.TESTPOINT 32.92,57.89 11.84,57.89 9.93,55.98 9.93,25.04 v9.55,24.66

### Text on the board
tPlace: 3V3 | GND | BTLDR_TX | BATT | !RESET | ADC7 | ADC6 | ADC5 | ADC4 | ADC3 | BTLDR_CTRL | BTLDR_RX | C0 | Brad / Campbell | 2014/06/04 | C1 | C2 | I2C_SDA | I2C_SCL | SPI_CLK | JTAG | BTLDR | SPI_MOSI | SPI_MISO | USB_VDD | USB_N | PWR | USB_P | ATUM / Breakout | A | UNUSED | TMS | TCK | TDO | B6 | B5 | B4 | B3 | RX | TX | USBGND | UART | 5V | PROG | RESET

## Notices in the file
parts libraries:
SparkFun: Licensing: CC v3.0 Share-Alike You are welcome to use this library for commercial purposes.
